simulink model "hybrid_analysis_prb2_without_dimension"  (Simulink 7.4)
settings: Solver=ode4  SolverMode=SingleTasking  StartTime=0.0  StopTime=60.0  FixedStep=0.0005  RelTol=1e-3
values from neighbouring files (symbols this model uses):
  AR1 = 1    [prb2.m]
  AR2 = 4.125    [prb2.m]
  AR3 = 1    [prb2.m]
  c1_mu1 = 1    [prb2.m]
  c1_mu2 = 1    [prb2.m]
  c2_mu1 = 0.1316    [prb2.m]
  c2_mu2 = 0.0001748    [prb2.m]
  c3_mu1 = 1    [prb2.m]
  c3_mu2 = 1    [prb2.m]
  Hf = 0.310    (= 0.31)    [prb2.m]
  Ici = 0.009020    (= 0.00902)    [prb2.m]
  Ici12 = It2 - It    (= 0.0149238079833)    [prb2.m]
  Icr = 0.005806    [prb2.m]
  Icr12 = Icr + Isi/(R1*R1) + Ici/(R2*R2)    (= 0.0366753653)    [prb2.m]
  Isi = 0.001020    (= 0.00102)    [prb2.m]
  Isi12 = It1 - It    (= 0.00429856082609)    [prb2.m]
  Isr = 1    [prb2.m]
  It = 0.05623    [prb2.m]
  It1 = It + Isi + R1*R1*Icr + R1*R1*Ici/(R2*R2)    (= 0.0605285608261)    [prb2.m]
  It2 = It + Ici + R2*R2*Icr + R2*R2*Isi/(R1*R1)    (= 0.0711538079833)    [prb2.m]
  Iwf = 2.8    [prb2.m]
  Ks = 6742.0    (= 6742)    [prb2.m]
  M = 1644.0 + 125.0    (= 1769)    [prb2.m]
  m_s_to_km_h = 3.6    [prb2.m]
  Pc1init = 0    [prb2.m]
  Pc1max = 1    [prb2.m]
  Pc2init = 0    [prb2.m]
  Pc2max = 400.0    (= 400)    [prb2.m]
  Pc3init = 0    [prb2.m]
  Pc3max = 1    [prb2.m]
  pres_index = [-5,5]    [prb2.m]
  R1 = Rci*Rsi/(1-Rci*Rcr)    (= 0.342353138929)    [prb2.m]
  R2 = Rci    (= 0.6379)    [prb2.m]
  R4 = 1    [prb2.m]
  Rci = 0.6379    [prb2.m]
  Rcr = 0.7045    [prb2.m]
  Rd = 0.3521    [prb2.m]
  Rr = 1    [prb2.m]
  Rsi = 0.2955    [prb2.m]
  Rsr = 1    [prb2.m]
  tau1off = 0    [prb2.m]
  tau1on = 1    [prb2.m]
  tau2off = 0    [prb2.m]
  tau2on = 1    [prb2.m]
  tau3off = 0    [prb2.m]
  tau3on = 1    [prb2.m]
  Ts_init = 0    [prb2.m]
  V_init = 0    [prb2.m]
  Wt_init = 0    [prb2.m]
undefined symbols (not defined in the file or in its folder): c1_table, c2_table, c3_table, shift_1_2, shift_2_1, trans, trans_v1_1
libraries: simulink x1
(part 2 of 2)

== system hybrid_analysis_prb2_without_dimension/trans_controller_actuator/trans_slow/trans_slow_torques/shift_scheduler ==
  note: References: - D. Cho and J.K. Hedrick: "Automotive Powertrain Modeling for Control", ASME Trans. V111, Dec. 1989, pp. 568-576. - Butts, K., "Analysis Needs for Automotive Powertrain Control," Proceedings of The 7th Mechatronics Forum International Conference, September 6-8 2000, Atlanta, Georgia.
  tps : Inport
  vss : Inport  Port=2
  p_e_switch : Inport  Port=3
  gear : Inport  Port=4
  1_2_shift : Lookup  InputValues=shift_1_2.x  Table=shift_1_2.y
  2_1_shift : Lookup  InputValues=shift_2_1.x  Table=shift_2_1.y
  Product : Product
  Product1 : Product
  Switch : Switch  Threshold=0.5
  economy : Constant  Value=0.75
  m_s_to_km_h : Gain  Gain=m_s_to_km_h
  power : Constant
  shift_schedule : Stateflow chart
  ngear : Outport  InitialOutput=0
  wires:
  shift_schedule/1(to_gear) -> ngear/1  "to_gear"
  gear/1 -> shift_schedule/1(gear)
  Switch/1 -> Product/2, Product1/2
  m_s_to_km_h/1 -> shift_schedule/2(V)  "vss_kmh"
  vss/1 -> m_s_to_km_h/1
  tps/1 -> 1_2_shift/1, 2_1_shift/1
  Product/1 -> shift_schedule/3(shift_speed_12)
  1_2_shift/1 -> Product/1  "shift_speed_12"
  power/1 -> Switch/1
  economy/1 -> Switch/3
  p_e_switch/1 -> Switch/2
  Product1/1 -> shift_schedule/4(shift_speed_21)
  2_1_shift/1 -> Product1/1  "shift_speed_21"

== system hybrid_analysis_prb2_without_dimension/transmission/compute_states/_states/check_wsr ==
  note: If fabs(wsr) < 0.5 set it equal to 0.0
  In1 : Inport
  Abs : Abs
  Constant : Constant  Value=0.5
  Constant1 : Constant  Value=0
  Relational Operator : RelationalOperator  Operator=<
  Switch : Switch  Threshold=0.5
  Out1 : Outport
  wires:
  Constant/1 -> Relational Operator/2
  Switch/1 -> Out1/1  "w_sr"
  Relational Operator/1 -> Switch/2
  Abs/1 -> Relational Operator/1
  Constant1/1 -> Switch/1
  In1/1 -> Abs/1, Switch/3

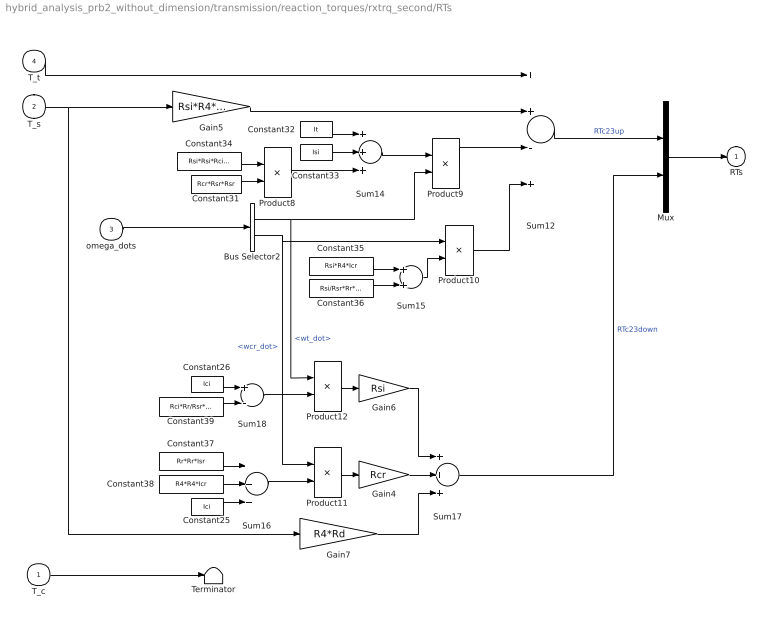
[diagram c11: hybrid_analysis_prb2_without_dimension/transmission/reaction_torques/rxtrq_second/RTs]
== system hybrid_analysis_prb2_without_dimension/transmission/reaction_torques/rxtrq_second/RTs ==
  T_c : Inport
  T_s : Inport  Port=2
  omega_dots : Inport  Port=3
  T_t : Inport  Port=4
  Bus Selector2 : BusSelector  OutputSignals=wt_dot,wcr_dot
  Constant25 : Constant  Value=Ici
  Constant26 : Constant  Value=Ici
  Constant31 : Constant  Value=Rcr*Rsr*Rsr
  Constant32 : Constant  Value=It
  Constant33 : Constant  Value=Isi
  Constant34 : Constant  Value=Rsi*Rsi*Rci*Isr
  Constant35 : Constant  Value=Rsi*R4*Icr
  Constant36 : Constant  Value=Rsi/Rsr*Rr*Isr
  Constant37 : Constant  Value=Rr*Rr*Isr
  Constant38 : Constant  Value=R4*R4*Icr
  Constant39 : Constant  Value=Rci*Rr/Rsr*Isr
  Gain4 : Gain  Gain=Rcr
  Gain5 : Gain  Gain=Rsi*R4*Rd
  Gain6 : Gain  Gain=Rsi
  Gain7 : Gain  Gain=R4*Rd
  Mux : Mux  Inputs=2
  Product{9..12} (4 alike) : Product
  Product8 : Product  Inputs=*/
  Sum12 : Sum  Inputs=++-+
  Sum14 : Sum  Inputs=+++
  Sum15 : Sum
  Sum16 : Sum  Inputs=+++
  Sum17 : Sum  Inputs=+++
  Sum18 : Sum  Inputs=+-
  Terminator : Terminator
  RTs : Outport  InitialOutput=[0,0,0]
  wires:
  T_t/1 -> Sum12/1
  Gain5/1 -> Sum12/2
  Constant31/1 -> Product8/2
  omega_dots/1 -> Bus Selector2/1
  Sum14/1 -> Product9/1
  Constant32/1 -> Sum14/1
  Product8/1 -> Sum14/3
  Constant33/1 -> Sum14/2
  Constant34/1 -> Product8/1
  Product9/1 -> Sum12/3
  Constant35/1 -> Sum15/1
  Constant36/1 -> Sum15/2
  Sum15/1 -> Product10/2
  Product10/1 -> Sum12/4
  Mux/1 -> RTs/1
  Sum12/1 -> Mux/1  "RTc23up"
  Bus Selector2/2 -> Product10/1, Product11/1  "<wcr_dot>"
  Bus Selector2/1 -> Product9/2, Product12/1  "<wt_dot>"
  T_s/1 -> Gain5/1, Gain7/1
  Gain7/1 -> Sum17/3
  Sum17/1 -> Mux/2  "RTc23down"
  T_c/1 -> Terminator/1
  Product11/1 -> Gain4/1
  Gain4/1 -> Sum17/2
  Sum16/1 -> Product11/2
  Product12/1 -> Gain6/1
  Gain6/1 -> Sum17/1
  Constant37/1 -> Sum16/1
  Constant38/1 -> Sum16/2
  Constant25/1 -> Sum16/3
  Constant26/1 -> Sum18/1
  Constant39/1 -> Sum18/2
  Sum18/1 -> Product12/2

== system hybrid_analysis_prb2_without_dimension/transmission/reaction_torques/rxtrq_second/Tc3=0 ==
  T_t : Inport
  omega_dots : Inport  Port=2
  T_s : Inport  Port=3
  T_c : Inport  Port=4
  Enable : EnablePort  StatesWhenEnabling=reset
  Bus Selector2 : BusSelector  OutputSignals=wt_dot,wsi_dot,wci_dot
  Constant24 : Constant  Value=It
  Constant25 : Constant  Value=Ici
  Gain : Gain  Gain=Isi/Rsi
  Gain1 : Gain  Gain=Rsr/Rci
  Gain2 : Gain  Gain=It
  Gain3 : Gain  Gain=Ici12
  Gain4 : Gain  Gain=Rd*R2
  Mux : Mux  Inputs=3
  Product6 : Product
  Sum10 : Sum  Inputs=+-
  Sum11 : Sum
  Sum2 : Sum  Inputs=+--
  Sum9 : Sum
  Terminator : Terminator
  RTs : Outport
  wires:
  omega_dots/1 -> Bus Selector2/1
  Constant24/1 -> Sum9/1
  Constant25/1 -> Sum9/2
  Sum9/1 -> Product6/1
  Product6/1 -> Sum2/2
  Gain/1 -> Sum2/3
  Sum2/1 -> Gain1/1
  Bus Selector2/1 -> Product6/2, Gain2/1  "<wt_dot>"
  Gain2/1 -> Sum10/2
  T_t/1 -> Sum2/1, Sum10/1
  Bus Selector2/2 -> Gain/1  "<wsi_dot>"
  Bus Selector2/3 -> Gain3/1  "<wci_dot>"
  Gain3/1 -> Sum11/1
  Gain1/1 -> Mux/1  "RTB12"
  Sum10/1 -> Mux/2  "RTc2up"
  Sum11/1 -> Mux/3  "RTc2down"
  Mux/1 -> RTs/1
  T_c/1 -> Terminator/1
  T_s/1 -> Gain4/1
  Gain4/1 -> Sum11/2

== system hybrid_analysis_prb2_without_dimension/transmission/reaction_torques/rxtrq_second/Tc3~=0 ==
  T_c : Inport
  T_s : Inport  Port=2
  omega_dots : Inport  Port=3
  T_t : Inport  Port=4
  Enable : EnablePort  StatesWhenEnabling=reset
  Bus Selector2 : BusSelector  OutputSignals=wsr_dot,wt_dot,wsi_dot,wci_dot,wcr_dot
  Bus Selector3 : BusSelector  OutputSignals=tc3
  Constant24 : Constant  Value=It
  Constant25 : Constant  Value=Ici
  Gain : Gain  Gain=Isi/Rsi
  Gain1 : Gain  Gain=Rsr/R2
  Gain2 : Gain  Gain=It
  Gain3 : Gain  Gain=Ici
  Gain4 : Gain  Gain=Rcr/Rsi
  Gain5 : Gain  Gain=Isr
  Gain6 : Gain  Gain=R2/R1
  Gain7 : Gain  Gain=R2/R1*Isi
  Gain8 : Gain  Gain=R2*Icr
  Gain9 : Gain  Gain=R2*Rd
  Mux : Mux  Inputs=3
  Product6 : Product
  Sum10 : Sum  Inputs=++-
  Sum11 : Sum  Inputs=+++++
  Sum12 : Sum
  Sum2 : Sum  Inputs=++--
  Sum9 : Sum
  RTs : Outport
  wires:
  omega_dots/1 -> Bus Selector2/1
  Constant24/1 -> Sum9/1
  Constant25/1 -> Sum9/2
  Sum9/1 -> Product6/1
  Bus Selector2/2 -> Product6/2, Gain2/1  "<wt_dot>"
  T_c/1 -> Bus Selector3/1
  Bus Selector3/1 -> Gain4/1, Sum10/2, Gain6/1  "<tc3>"
  Product6/1 -> Sum2/3
  Gain/1 -> Sum2/4
  Sum2/1 -> Gain1/1
  Gain2/1 -> Sum10/3
  Sum10/1 -> Mux/2  "RTc2up"
  Gain4/1 -> Sum2/1
  Gain1/1 -> Sum12/2
  Sum12/1 -> Mux/1  "RTB12"
  Gain5/1 -> Sum12/1
  Bus Selector2/1 -> Gain5/1  "<wsr_dot>"
  T_t/1 -> Sum2/2, Sum10/1
  Mux/1 -> RTs/1
  Bus Selector2/3 -> Gain/1, Gain7/1  "<wsi_dot>"
  Bus Selector2/4 -> Gain3/1  "<wci_dot>"
  Sum11/1 -> Mux/3  "RTc2down"
  Bus Selector2/5 -> Gain8/1  "<wcr_dot>"
  T_s/1 -> Gain9/1
  Gain3/1 -> Sum11/1
  Gain9/1 -> Sum11/2
  Gain6/1 -> Sum11/3
  Gain7/1 -> Sum11/4
  Gain8/1 -> Sum11/5

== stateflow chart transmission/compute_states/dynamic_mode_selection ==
  state engaged
    state first
      entry:
      first=true;
      mode_select=1;
      a_gear=1
      exit:
      first=false;
    state shift121
      state torque121
        entry:
        torque121=true;
        mode_select=2;
        a_gear=1.5;
        exit:
        torque121=false;
      state inertia121
        entry:
        inertia121=true;
        mode_select=3;
        exit:
        inertia121=false;
      (default) -> torque121
      torque121 -> inertia121 : [c1slip ~= 0 || ... RTsp1 ~= 0 && c1slip==0]
    state second
      entry:
      second=true;
      mode_select=4;
      a_gear=2
      exit:
      second=false;
    (default) -> first
    inertia121 -> first : [Tc1 > Tt && c1slip ==0 && w_sr ==0]
    first -> shift121 : [Tc2 > 0 && RTsp1<=0]
    inertia121 -> second : [(c2slip == 0.0) && ( ( (fabs(Tc2) > fabs(RTc2up)) && (fabs(Tc2) > fabs(RTc2down)) ) || ...  ( (fabs(Tc2) > fabs(RTc23up)) && (fabs(Tc2) > fabs(RTc23down)) ) || ...  ( (fabs(Tc2) > fabs(RTc24up)) && (fabs(Tc2) > fabs(RTc24down)) ) )]
    second -> shift121 : [!((c2slip == 0.0) && ( ( (fabs(Tc2) > fabs(RTc2up)) && (fabs(Tc2) > fabs(RTc2down)) ) || ...  ( (fabs(Tc2) > fabs(RTc23up)) && (fabs(Tc2) > fabs(RTc23down)) ) || ...  ( (fabs(Tc2) > fabs(RTc24up)) && (fabs(Tc2) > fabs(RTc24down)) ) ))]
  (default) -> engaged

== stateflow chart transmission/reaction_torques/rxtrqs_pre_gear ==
  state second_gear
    entry:do_rxtrq_second=true;
    exit:do_rxtrq_second=false;
  state first_gear
    entry:do_rxtrq_first=true;
    exit:do_rxtrq_first=false;
  state shift121
    entry:do_rxtrq_shift121=true;
    exit:do_rxtrq_shift121=false;
  (default) -> first_gear
  shift121 -> second_gear : [gear==2]
  second_gear -> shift121 : [gear==1.5]
  first_gear -> shift121 : [gear==1.5]
  shift121 -> first_gear : [gear==1]

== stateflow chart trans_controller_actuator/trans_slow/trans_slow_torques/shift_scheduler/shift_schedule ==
  state first_gear
    entry: to_gear = 1;
  state transition12
    state shifting
      entry: to_gear=2;
    state shift_pending
      entry: ctr=0;
      to_gear=1;
      during: ctr=ctr+1;
    shift_pending -> shifting : [ctr > DELAY]
  state transition21
    state shift_pending
      entry: ctr=0;
      to_gear=2;
      during: ctr = ctr+1;
    state shifting
      entry: to_gear=1;
    shift_pending -> shifting : [ctr > DELAY]
  state second_gear
    entry: to_gear=2;
  (default) -> first_gear
  transition21 -> second_gear : [V > shift_speed_12]
  second_gear -> shift_pending : [V <= shift_speed_21]
  shifting -> first_gear : [gear == 1]
  shifting -> second_gear : [gear == 2]
  transition12 -> first_gear : [V <= shift_speed_21]
  first_gear -> shift_pending : [V > shift_speed_12]

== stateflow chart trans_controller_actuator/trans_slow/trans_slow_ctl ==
  (default) -> (junction 83)
  (junction 83) -> (junction 84) : time_slow{do_trans_slow_torques;t;}
